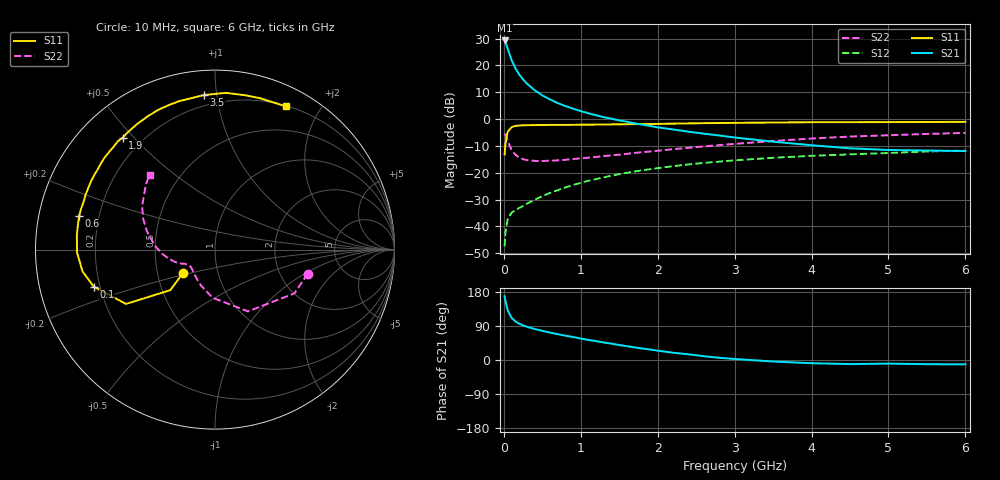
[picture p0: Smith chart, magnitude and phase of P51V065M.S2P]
! SIEMENS Small Signal Semiconductors
! BFP183
! Si NPN RF Bipolar Junction Transistor in SOT143
! VCE = 1 V  IC = 65 mA
! Common Emitter S-Parameters:  March  1996
# GHz  S  MA  R  50
!  f  S11  S21  S12  S22
! GHz  MAG  ANG  MAG  ANG  MAG  ANG  MAG  ANG
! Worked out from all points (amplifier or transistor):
!   36 points, 10 MHz to 6 GHz, reference 50 ohm
!   highest |S21| = 29.3 dB at 10 MHz (marker M1)
!   |S21| within 3 dB of that: start of sweep to 49.39 MHz
!   unconditionally stable (mu >= 1): start of sweep to 45.59 MHz; 92.52 MHz to end of sweep
!   at 250 MHz: K = 1.55, MAG = 19.2 dB, |S12| = -32.4 dB
!   at 1.4 GHz: K = 2.06, MAG = 4.7 dB, |S12| = -21.1 dB
!   at 6 GHz: K = 1.59, MAG = -4.6 dB, |S12| = -11.7 dB
!   S11 on the Smith chart (normalised r, x): 10 MHz: 0.68, -0.18; 100 MHz: 0.18, -0.14; 600 MHz: 0.13, +0.12; 1.9 GHz: 0.13, +0.47; 3.5 GHz: 0.14, +0.92; 6 GHz: 0.21, +1.59
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0.01  0.2203 -143.9  29.16 168.0  0.0043 58.3  0.5339 -14.5
0.02  0.3363 -137.8  27.57 156.5  0.0076 60.2  0.5052 -28.9
0.05  0.5811 -148.6  20.52 131.3  0.0137 48.2  0.3902 -61.9
0.1  0.7062 -163.0  12.62 111.5  0.018 39.8  0.2687 -92.8
0.15  0.7484 -170.7  8.875 101.8  0.0203 40.0  0.2166 -110.5
0.2  0.758 -175.4  6.778 95.8  0.0222 43.2  0.1924 -121.8
0.25  0.7693 -178.9  5.476 91.3  0.0241 45.3  0.1797 -129.2
0.3  0.7691 178.4  4.58 87.7  0.0266 48.9  0.1719 -135.0
0.4  0.7739 174.0  3.456 81.8  0.0314 53.7  0.1666 -142.0
0.5  0.7758 170.2  2.767 77.0  0.0367 55.7  0.1661 -146.3
0.6  0.78 166.1  2.328 72.3  0.0423 57.5  0.1676 -148.9
0.7  0.7802 163.0  1.987 68.2  0.0475 58.9  0.1704 -150.8
0.8  0.7791 159.9  1.749 64.2  0.0533 59.7  0.1746 -152.1
1.1  0.7888 151.0  1.282 52.9  0.0711 59.4  0.1915 -155.7
1.5  0.8007 140.3  0.946 39.4  0.0942 56.8  0.2176 -160.4
1.9  0.8082 129.5  0.746 27.7  0.1167 52.3  0.2494 -166.5
2.2  0.8232 121.9  0.641 19.2  0.1328 48.8  0.2752 -171.7
2.8  0.8452 107.7  0.495 5.8  0.1616 40.8  0.328 177.7
3.5  0.8635 94.0  0.38 -4.0  0.1903 32.1  0.3913 165.2
4.5  0.8762 78.9  0.286 -10.8  0.2203 20.1  0.4727 149.2
5.5  0.8822 68.3  0.26 -11.1  0.2491 9.9  0.5295 136.7
6  0.8897 63.7  0.254 -11.5  0.2587 4.6  0.5536 131.2
